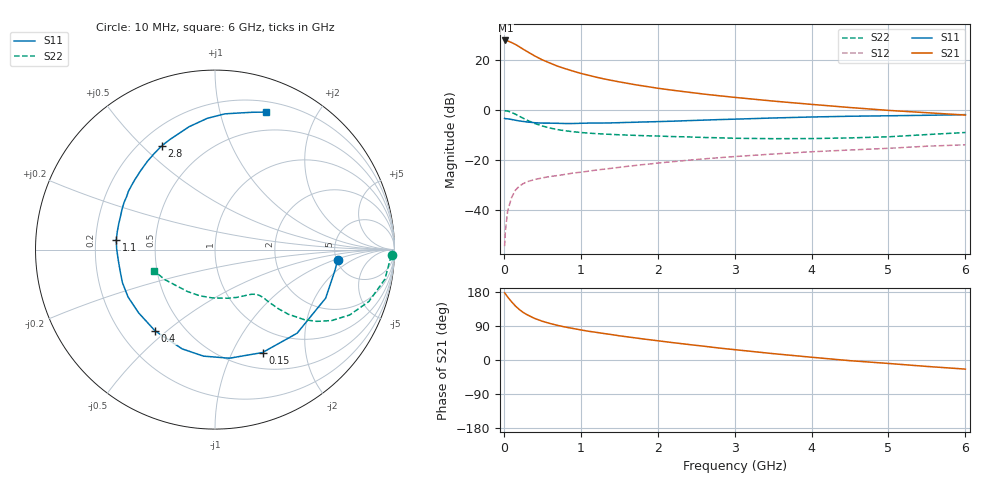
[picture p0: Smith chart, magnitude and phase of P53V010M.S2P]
! SIEMENS Small Signal Semiconductors
! BFP183
! Si NPN RF Bipolar Junction Transistor in SOT143
! VCE = 3 V  IC = 10 mA
! Common Emitter S-Parameters:  March  1996
# GHz  S  MA  R  50
!  f  S11  S21  S12  S22
! GHz  MAG  ANG  MAG  ANG  MAG  ANG  MAG  ANG
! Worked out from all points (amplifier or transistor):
!   36 points, 10 MHz to 6 GHz, reference 50 ohm
!   highest |S21| = 27.9 dB at 20 MHz (marker M1)
!   |S21| within 3 dB of that: start of sweep to 225.6 MHz
!   unconditionally stable (mu >= 1): 1.171 GHz to 5.572 GHz
!   at 250 MHz: K = 0.32, MSG = 26.9 dB, |S12| = -29.4 dB
!   at 1.4 GHz: K = 1.08, MAG = 15.9 dB, |S12| = -23.2 dB
!   at 6 GHz: K = 0.94, MSG = 6.0 dB, |S12| = -13.8 dB
!   lowest NFmin = 1.30 dB at 450 MHz
!   S11 on the Smith chart (normalised r, x): 10 MHz: 5.12, -1.09; 150 MHz: 0.69, -1.32; 400 MHz: 0.34, -0.46; 1.1 GHz: 0.29, +0.05; 2.8 GHz: 0.29, +0.57; 6 GHz: 0.30, +1.39
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0.01  0.6855 -4.7  24.89 177.2  0.0019 81.7  0.9847 -1.9
0.02  0.6786 -9.6  24.94 174.8  0.0038 85.6  0.975 -3.9
0.05  0.6733 -23.7  24.41 166.2  0.0097 81.0  0.9614 -9.8
0.1  0.6529 -45.5  22.67 153.8  0.0178 69.9  0.905 -18.6
0.15  0.6317 -65.2  20.77 142.6  0.025 61.0  0.834 -25.9
0.2  0.6105 -82.4  18.72 133.4  0.0302 56.3  0.761 -31.3
0.25  0.597 -96.1  16.71 125.7  0.0338 51.1  0.6935 -35.2
0.3  0.5827 -108.3  15.06 119.7  0.037 48.1  0.6331 -38.1
0.4  0.5626 -126.4  12.25 109.7  0.041 44.6  0.5445 -41.4
0.5  0.5525 -140.3  10.2 102.3  0.0442 42.3  0.484 -43.0
0.6  0.5518 -151.4  8.798 96.4  0.0471 41.3  0.4405 -43.8
0.7  0.5476 -160.4  7.605 91.3  0.0493 41.5  0.4092 -44.4
0.9  0.5423 -174.1  6.071 83.2  0.0552 41.5  0.3713 -45.2
1.1  0.5528 174.3  5.017 75.9  0.0603 42.4  0.3483 -46.5
1.5  0.5636 157.1  3.7 63.9  0.0718 43.6  0.3227 -50.4
1.8  0.5816 146.0  3.082 55.8  0.0814 43.4  0.3102 -54.8
2.2  0.6038 133.4  2.508 45.7  0.0935 42.5  0.2969 -61.8
2.8  0.6501 117.1  1.949 31.5  0.1122 39.3  0.2808 -74.8
3.5  0.6997 101.9  1.526 16.8  0.1328 35.2  0.2696 -93.2
4.5  0.7582 85.9  1.133 -1.8  0.1599 27.9  0.2793 -123.3
5.5  0.7928 74.8  0.892 -17.0  0.1905 21.1  0.3257 -149.1
6  0.8164 69.8  0.801 -24.0  0.2034 16.7  0.3584 -160.5
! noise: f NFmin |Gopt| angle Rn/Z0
0.45  1.3  0.15  45  0.18
0.9  1.4  0.2  125  0.19
1.8  2.1  0.34  -170  0.14
